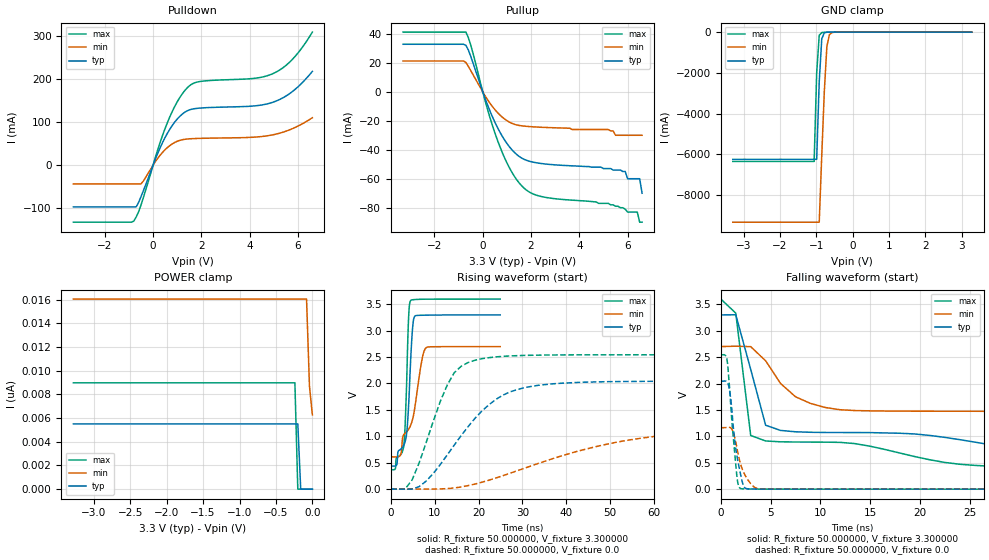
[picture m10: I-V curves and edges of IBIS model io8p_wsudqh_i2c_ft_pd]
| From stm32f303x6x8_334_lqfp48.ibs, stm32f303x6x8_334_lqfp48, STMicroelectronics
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|   Model io8p_wsudqh_i2c_ft_pd
[Model]  io8p_wsudqh_i2c_ft_pd
Model_type I/O
Polarity   Non-Inverting
Enable   Active-Low
Vinl =   0.990000V
Vinh =   2.310000V
Vmeas =  1.650000V
Cref =   30.000000pF
Rref =   100.000000M
Vref =   0.0V
C_comp   0.0F   0.0F   0.0F
[Temperature Range]   25.000000   0.140000k   -40.000000
[Pullup Reference]   3.300000V   2.700000V   3.600000V
[Pulldown Reference]   0.0V   0.0V   0.0V
[POWER Clamp Reference]   3.300000V   2.700000V   3.600000V
[GND Clamp Reference]   0.0V   0.0V   0.0V
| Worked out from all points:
|   slope of the pulldown table from 0 to 0.495 V, typ, clamps not added: 7.75 ohm
|   slope of the pullup table from 0 to 0.495 V, typ, clamps not added: 23.9 ohm
|   GND clamp passes 1 mA (typ) near -0.60 V on its own axis
|   rising waveform, R_fixture 50.000000, V_fixture 3.300000: 20-80 % time 1.17ns typ, 3.83ns min, 775ps max; typ from 0.435 V to 3.3 V
|   rising waveform, R_fixture 50.000000, V_fixture 0.0: 20-80 % time 12.2ns typ, 29.8ns min, 6.8ns max; typ from 0 V to 2.04 V
|   falling waveform, R_fixture 50.000000, V_fixture 3.300000: 20-80 % time 19.1ns typ, 55.7ns min, 1.31ns max; typ from 3.3 V to 0.435 V
|   falling waveform, R_fixture 50.000000, V_fixture 0.0: 20-80 % time 803ps typ, 1.07ns min, 653ps max; typ from 2.04 V to 0 V
[Pulldown]
|Voltage   I(typ)   I(min)   I(max)
-3.3V     -96.32mA   -43.01mA   -131.7mA
-800mV    -96.32mA   -43.01mA   -129.4mA
-700mV    -96.32mA   -43.01mA   -120mA
-500mV    -72.9mA    -43.01mA   -92.16mA
200mV     28.44mA    16.57mA    37.01mA
600mV     74.69mA    41.37mA    99.56mA
1V        107mA      55.62mA    146.8mA
1.4V      125.8mA    60.81mA    178.5mA
1.9V      132.3mA    62.32mA    193.7mA
5V        146.7mA    71.07mA    213.2mA
5.8V      172.1mA    85.55mA    247mA
6.6V      217.6mA    110.2mA    308.5mA
[Pullup]
|Voltage   I(typ)   I(min)   I(max)
-3.3V     32.82mA    21.28mA    41.22mA
-700mV    32.15mA    20.32mA    41.22mA
700mV     -27.48mA   -15.83mA   -37.39mA
1.2V      -39.86mA   -21.71mA   -55.32mA
1.8V      -47.22mA   -23.81mA   -67.73mA
5.2V      -53mA      -26mA      -77mA
5.7V      -54mA      -30mA      -80mA
5.9V      -55mA      -30mA      -81mA
6V        -60mA      -30mA      -83mA
6.4V      -60mA      -30mA      -83mA
6.5V      -60mA      -30mA      -90mA
6.6V      -70mA      -30mA      -90mA
[GND_clamp]
|Voltage   I(typ)   I(min)   I(max)
-3.3V     -6.241A    -9.325A    -6.345A
-1.06V    -6.241A    -9.325A    -6.345A
-990mV    -6.241A    -9.325A    -2.007A
-920mV    -2.435A    -9.325A    -157.2mA
-850mV    -331.2mA   -6.034A    -23.12mA
-780mV    -36.14mA   -2.918A    -12.66mA
-710mV    -6.451mA   -709.1mA   -7.399mA
-640mV    -1.635mA   -128.1mA   -3.362mA
-570mV    -385.3uA   -25.27mA   -968.5uA
3.28V     78.94uA    62.35uA    85.92uA
[POWER_clamp]
|Voltage   I(typ)   I(min)   I(max)
-3.28V    5.515nA    16.06nA    8.985nA
-240mV    5.515nA    16.06nA    8.985nA
-200mV    5.515nA    16.06nA    0A
-160mV    0A         16.06nA    0A
-80mV     0A         16.06nA    0A
-40mV     0A         8.703nA    0A
0V        0A         6.282nA    0A
[Ramp]
| variable   typ   min   max
dV/dt_r  1.22556/12.15514n   0.69816/29.72013n   1.52568/6.74861n
dV/dt_f  1.71839/18.79800n   1.25302/55.57922n   1.94023/1.25723n
R_load = 50.000000
[Rising Waveform]
R_fixture= 50.000000
V_fixture= 3.300000
V_fixture_min= 2.700000
V_fixture_max= 3.600000
|time   V(typ)   V(min)   V(max)
0s        434.8mV    609mV      365.2mV
2.102ns   747.9mV    638.2mV    642.4mV
2.903ns   831.9mV    1.03V      825.4mV
3.253ns   913.5mV    1.059V     1.315V
3.654ns   1.142V     1.093V     2.346V
4.004ns   1.594V     1.133V     3.259V
4.404ns   2.338V     1.196V     3.563V
5.205ns   3.239V     1.436V     3.588V
8.108ns   3.294V     2.683V     3.596V
24.92ns   3.299V     2.699V     3.599V
[Rising Waveform]
R_fixture= 50.000000
V_fixture= 0.0
V_fixture_min= 0.0
V_fixture_max= 0.0
|time   V(typ)   V(min)   V(max)
0s        1.109nV    13.68nV    939.4pV
3.203ns   -1.36mV    -684.2uV   562.5uV
4.805ns   -1.496mV   -965.4uV   172.7mV
11.21ns   461.3mV    1.516mV    1.654V
14.41ns   830.9mV    18.95mV    2.202V
20.82ns   1.485V     130.3mV    2.471V
28.83ns   1.883V     345.9mV    2.527V
56.06ns   2.038V     949.7mV    2.543V
96.1ns    2.043V     1.146V     2.543V
797.6ns   2.043V     1.164V     2.543V
[Falling Waveform]
R_fixture= 50.000000
V_fixture= 3.300000
V_fixture_min= 2.700000
V_fixture_max= 3.600000
|time   V(typ)   V(min)   V(max)
0s        3.299V     2.699V     3.599V
1.502ns   3.302V     2.707V     3.333V
3.003ns   2.268V     2.698V     1.016V
4.505ns   1.21V      2.43V      912.7mV
6.006ns   1.112V     2V         896.6mV
12.01ns   1.072V     1.503V     885.9mV
33.03ns   659.5mV    1.461V     401mV
75.08ns   448.5mV    808.1mV    366.7mV
114.1ns   437.1mV    656.9mV    365.3mV
747.7ns   434.8mV    609mV      365.2mV
[Falling Waveform]
R_fixture= 50.000000
V_fixture= 0.0
V_fixture_min= 0.0
V_fixture_max= 0.0
|time   V(typ)   V(min)   V(max)
0s        2.043V     1.164V     2.543V
600.6ps   2.035V     1.17V      2.474V
700.7ps   2.008V     1.172V     2.346V
1.001ns   1.708V     1.159V     1.571V
1.301ns   1.084V     1.05V      881.5mV
1.602ns   650.4mV    798.1mV    265mV
2.002ns   264.3mV    462.6mV    10.67mV
2.402ns   27.15mV    277mV      4.63mV
3.904ns   2.28mV     6.306mV    1.815mV
49.85ns   1.109nV    13.68nV    939.4pV
